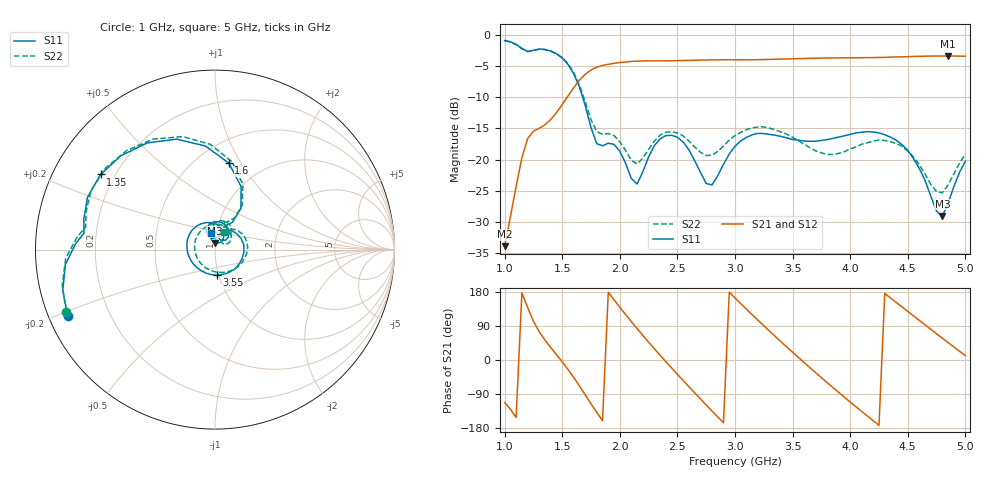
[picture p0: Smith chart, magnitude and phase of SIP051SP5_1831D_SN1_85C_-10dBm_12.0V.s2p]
# GHz  S  dB  R  50
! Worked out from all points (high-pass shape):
!   81 points, 1 GHz to 5 GHz, reference 50 ohm
!   highest |S21| = -3.40 dB at 4.85 GHz (marker M1); lowest = -33.9 dB at 1 GHz (marker M2)
!   |S21| within 3 dB of the highest: 1.696 GHz to end of sweep
!   lowest |S11| = -29.0 dB at 4.8 GHz (marker M3), VSWR 1.07, Z = 49.8 + j3.53 ohm
!   |S11| at or under -10 dB: 1.677 GHz to end of sweep
!   |S22| runs from -25.3 to -0.9 dB; largest |S21 - S12| = 0.002
!   S11 on the Smith chart (normalised r, x): 1 GHz: 0.06, -0.21; 1.35 GHz: 0.15, +0.29; 1.6 GHz: 0.70, +0.89; 3.55 GHz: 0.98, -0.29; 5 GHz: 0.94, +0.18
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1  -0.92 -155.7  -33.85 -112.6  -33.98 -111.7  -0.93 -157.3
1.2  -2.67 172.8  -16.63 138.4  -16.63 138.3  -2.71 170.0
1.35  -2.35 146.7  -14.42 52.8  -14.42 52.7  -2.38 143.5
1.6  -6.24 80.9  -8.46 -46.1  -8.45 -46.2  -6.05 79.0
1.7  -11.33 57.8  -6.32 -92.2  -6.31 -92.2  -10.73 58.5
1.85  -17.78 81.7  -4.92 -160.2  -4.91 -160.2  -15.93 73.9
1.95  -17.55 78.4  -4.58 158.8  -4.58 158.8  -16.16 70.6
2.15  -23.91 100.0  -4.23 82.9  -4.21 83.0  -20.70 82.1
2.35  -16.66 101.5  -4.18 12.4  -4.16 12.5  -16.05 85.7
2.5  -16.41 68.3  -4.16 -37.7  -4.14 -37.7  -15.73 61.4
2.65  -20.16 43.0  -4.08 -86.5  -4.06 -86.5  -17.97 46.7
2.8  -24.06 65.7  -4.02 -134.4  -4.00 -134.5  -19.27 54.4
3  -17.85 58.2  -4.01 163.8  -4.00 163.7  -16.14 46.3
3.25  -15.82 -3.7  -3.98 90.3  -3.97 90.4  -14.76 4.3
3.55  -16.87 -86.1  -3.82 6.8  -3.81 6.8  -16.97 -60.5
3.7  -17.05 -123.7  -3.75 -33.5  -3.75 -33.5  -18.60 -104.0
4  -15.96 170.2  -3.70 -110.9  -3.69 -110.9  -18.29 154.1
4.35  -16.39 98.0  -3.58 163.7  -3.60 163.7  -17.12 66.7
4.6  -21.40 55.3  -3.46 104.5  -3.45 104.4  -20.81 27.1
4.8  -29.03 90.6  -3.41 57.5  -3.39 57.6  -25.30 49.6
4.85  -26.96 106.6  -3.40 45.9  -3.40 46.0  -24.02 60.2
5  -20.24 101.8  -3.44 11.5  -3.44 11.4  -19.08 61.7
